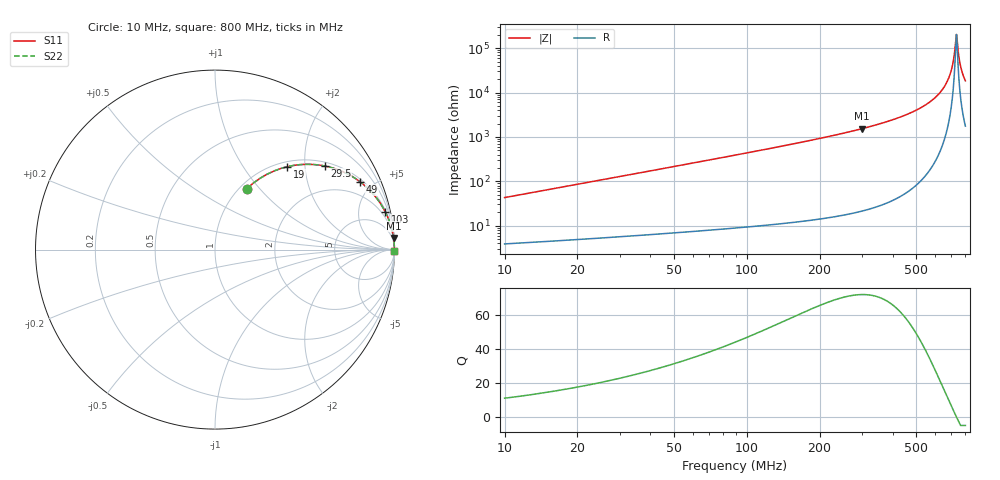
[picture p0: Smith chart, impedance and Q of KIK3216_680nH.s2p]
!version-2
!date-01.2022
!Series
# MHz S RI R 50
!Freq ReS11 ImS11 ReS21 ImS21 ReS12 ImS12 ReS22 ImS22
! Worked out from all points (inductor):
!   528 points, 10 MHz to 800 MHz, reference 50 ohm
!   read as one part in series: L = 680 nH near 13 MHz
!   highest Q = 72 at 298 MHz (marker M1), where L = 814 nH
!   self-resonance near 734.5 MHz
!   S11 on the Smith chart (normalised r, x): 10 MHz: 1.08, +0.85; 19 MHz: 1.10, +1.62; 29.5 MHz: 1.11, +2.52; 49 MHz: 1.14, +4.21; 103 MHz: 1.19, +8.98; 800 MHz: open
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10  0.1767 0.3387  0.8233 -0.3387  0.8233 -0.3387  0.1767 0.3387
19  0.4039 0.4621  0.5961 -0.4621  0.5961 -0.4621  0.4039 0.4621
29.5  0.6102 0.4661  0.3898 -0.4661  0.3898 -0.4661  0.6102 0.4661
49  0.808 0.378  0.192 -0.378  0.192 -0.378  0.808 0.378
103  0.9487 0.2103  0.0513 -0.2103  0.0513 -0.2103  0.9487 0.2103
142  0.9728 0.1539  0.0272 -0.1539  0.0272 -0.1539  0.9728 0.1539
274  0.9936 0.073  0.00639 -0.073  0.00639 -0.073  0.9936 0.073
298  0.9948 0.0652  0.00518 -0.0652  0.00518 -0.0652  0.9948 0.0652
406  0.9978 0.0399  0.00221 -0.0399  0.00221 -0.0399  0.9978 0.0399
538  0.9991 0.0201  0.000894 -0.0201  0.000894 -0.0201  0.9991 0.0201
614.5  0.9994 0.0114  0.000601 -0.0114  0.000601 -0.0114  0.9994 0.0114
668.5  0.9995 0.00602  0.00051 -0.00602  0.00051 -0.00602  0.9995 0.00602
691  0.9995 0.00391  0.000493 -0.00391  0.000493 -0.00391  0.9995 0.00391
709  0.9995 0.00227  0.000487 -0.00227  0.000487 -0.00227  0.9995 0.00227
719.5  0.9995 0.00134  0.000487 -0.00134  0.000487 -0.00134  0.9995 0.00134
731.5  0.9995 0.000284  0.000489 -0.000284  0.000489 -0.000284  0.9995 0.000284
734.5  0.9995 2.31e-05  0.00049 -2.31e-05  0.00049 -2.31e-05  0.9995 2.31e-05
737.5  0.9995 -0.000236  0.000491 0.000236  0.000491 0.000236  0.9995 -0.000236
751  0.9995 -0.00139  0.000498 0.00139  0.000498 0.00139  0.9995 -0.00139
761.5  0.9995 -0.00227  0.000506 0.00227  0.000506 0.00227  0.9995 -0.00227
778  0.9995 -0.00364  0.000521 0.00364  0.000521 0.00364  0.9995 -0.00364
800  0.9995 -0.00542  0.000548 0.00542  0.000548 0.00542  0.9995 -0.00542
